(* Logix 5000 Program export KEP; software revision 30.00; part 10 of 15 *)

ADD_ON_INSTRUCTION L_CLR   (* revision 1.0 20170709, vendor Ken Fischer, NSWCPD, C516 *)
// CLR (64-bit)
// Revision note:
// Initial Release
// Help:
// Adds two LINT (signed 64-bit) values and returns a LINT (signed 64-bit) sum.
// Also provides math status bits for Carry, Negative, Overflow and Zero result
// (equivalent to built-in S:C, S:N, S:V, S:Z).
VAR_IN_OUT
   Out : LINT; {required}   // Sum, 64-bit Integer
END_VAR
VAR
   Wrk : DINT[2];   // Input A as two 32-bit DINTs
END_VAR

ROUTINE Logic   (* ladder *)
// Do 64-bit addition
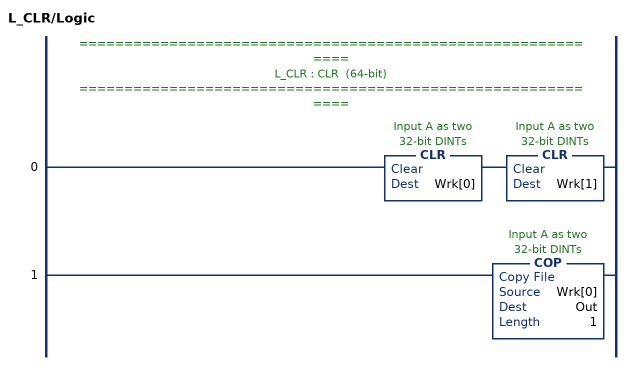
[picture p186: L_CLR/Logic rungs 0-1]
   // ============================================================
   // L_CLR : CLR  (64-bit)
   // ============================================================
   0: CLR(Wrk[0])CLR(Wrk[1]);
   1: COP(Wrk[0],Out,1);
END_ROUTINE
END_ADD_ON_INSTRUCTION

ADD_ON_INSTRUCTION L_EQU   (* revision 1.0 01 Release, vendor Rockwell Automation, ExecuteEnableInFalse *)
// Equal (64-bit)
// Revision note:
// Deleted unused Local Tag
// Help:
// This instruction compares two LINT (64-bit signed integer) variables.
// If Inp_A is equal to Inp_B, EnableOut and Out are set to true (1).
// Otherwise EnableOut and Out are cleared to false (0).
VAR_IN_OUT
   Inp_A : LINT; {required}   // Input A
   Inp_B : LINT; {required}   // Input B
END_VAR
VAR_OUTPUT
   Out : BOOL; {access Read Only, visible}   // TRUE if Inp_A is greater than or equal to Inp_B
END_VAR
VAR
   Wrk_Inp_B : DINT[2];   // 32-bit portions of Input B
   Wrk_Inp_A : DINT[2];   // 32-bit portions of Input A
END_VAR

ROUTINE EnableInFalse   (* ladder *)
// If rung is false, clear output "Out"
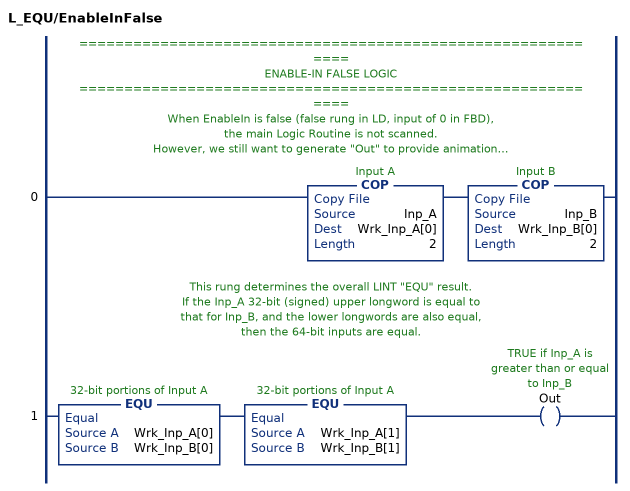
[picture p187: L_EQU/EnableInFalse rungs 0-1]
   // ============================================================
   // ENABLE-IN FALSE LOGIC
   // ============================================================
   // When EnableIn is false (false rung in LD, input of 0 in FBD),
   // the main Logic Routine is not scanned.
   // However, we still want to generate "Out" to provide animation!
   // ===================================================
   // CONVERT LINTs TO DINTs
   // ===================================================
   // These COPies take the input LINTs and break them into a
   // pair of DINTs each.  If the corresponding DINTs (high-order and high-order,
   // and low-order and low-order) are equal, then the input LINTs are equal.
   0: COP(Inp_A,Wrk_Inp_A[0],2)COP(Inp_B,Wrk_Inp_B[0],2);
   // This rung determines the overall LINT "EQU" result.
   // If the Inp_A 32-bit (signed) upper longword is equal to
   // that for Inp_B, and the lower longwords are also equal,
   // then the 64-bit inputs are equal.
   1: EQU(Wrk_Inp_A[0],Wrk_Inp_B[0])EQU(Wrk_Inp_A[1],Wrk_Inp_B[1])OTE(Out);
END_ROUTINE

ROUTINE Logic   (* ladder *)
// Compare inputs and output TRUE if they are equal
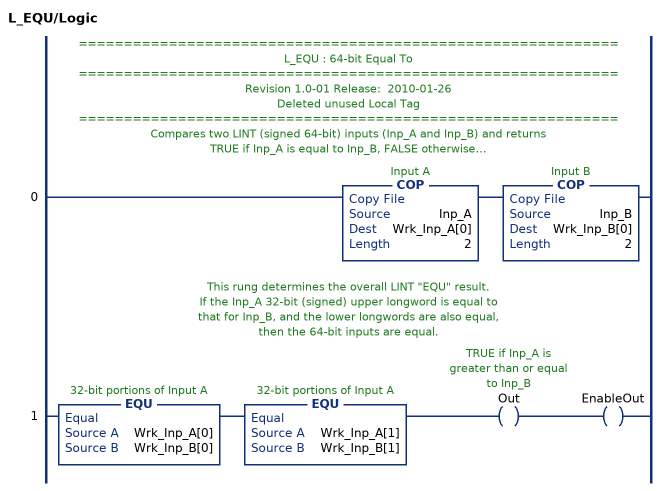
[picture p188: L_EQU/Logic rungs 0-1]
   // ============================================================
   // L_EQU : 64-bit Equal To
   // ============================================================
   // Revision 1.0-01 Release:  2010-01-26
   // Deleted unused Local Tag
   // ============================================================
   // Compares two LINT (signed 64-bit) inputs (Inp_A and Inp_B) and returns
   // TRUE if Inp_A is equal to Inp_B, FALSE otherwise.
   // This instruction breaks each LINT inputs into two DINTs
   // (32 bit signed each) to do the comparison.
   // ===================================================
   // CONVERT LINTs TO DINTs
   // ===================================================
   // These COPies take the input LINTs and break them into a
   // pair of DINTs each.  If the corresponding DINTs (high-order and high-order,
   // and low-order and low-order) are equal, then the input LINTs are equal.
   0: COP(Inp_A,Wrk_Inp_A[0],2)COP(Inp_B,Wrk_Inp_B[0],2);
   // This rung determines the overall LINT "EQU" result.
   // If the Inp_A 32-bit (signed) upper longword is equal to
   // that for Inp_B, and the lower longwords are also equal,
   // then the 64-bit inputs are equal.
   1: EQU(Wrk_Inp_A[0],Wrk_Inp_B[0])EQU(Wrk_Inp_A[1],Wrk_Inp_B[1])OTE(Out)OTE(EnableOut);
END_ROUTINE
END_ADD_ON_INSTRUCTION

ADD_ON_INSTRUCTION L_LES   (* revision 1.1 20170624, vendor Ken Fischer, NSWCPD, C516, ExecuteEnableInFalse *)
// Less Than (64-bit)
// Revision note:
// Rev1.1:  20170624 - Corrected comment on the Out bit
// Help:
// This instruction compares two LINT (64-bit signed integer) variables.
// If Inp_A is less than Inp_B, EnableOut and Out are set to true (1).
// Otherwise EnableOut and Out are cleared to false (0).
VAR_IN_OUT
   Inp_A : LINT; {required}   // Input A
   Inp_B : LINT; {required}   // Input B
END_VAR
VAR_OUTPUT
   Out : BOOL; {access Read Only, visible}   // TRUE if Inp_A is less than Inp_B
END_VAR
VAR
   Wrk_Inp_B : DINT[4];   // 32-bit portions of Input B
   Wrk_Inp_A : DINT[4];   // 32-bit portions of Input A
END_VAR

ROUTINE EnableInFalse   (* ladder *)
// If rung is false, clear output "Out"
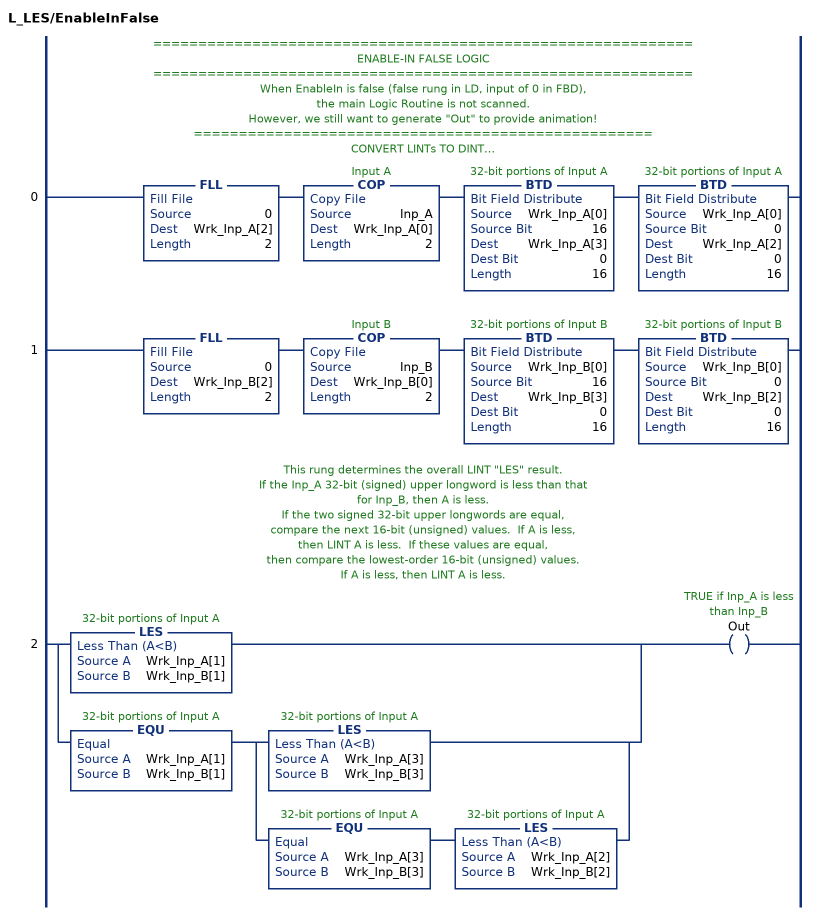
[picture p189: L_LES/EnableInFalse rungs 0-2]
   // ============================================================
   // ENABLE-IN FALSE LOGIC
   // ============================================================
   // When EnableIn is false (false rung in LD, input of 0 in FBD),
   // the main Logic Routine is not scanned.
   // However, we still want to generate "Out" to provide animation!
   // ===================================================
   // CONVERT LINTs TO DINTs
   // ===================================================
   // These COPies and BTDs take the input LINTs and break them into a
   // pair of DINTs each, then take the low-order signed DINT and breaks it
   // further into two 16-bit values so we can do unsigned compares on them.
   // Logix V17 has a LINT data type, but math instructions
   // (and AOI Input and Output Parameters) don't support LINT.
   0: FLL(0,Wrk_Inp_A[2],2)COP(Inp_A,Wrk_Inp_A[0],2)BTD(Wrk_Inp_A[0],16,Wrk_Inp_A[3],0,16)BTD(Wrk_Inp_A[0],0,Wrk_Inp_A[2],0,16);
   1: FLL(0,Wrk_Inp_B[2],2)COP(Inp_B,Wrk_Inp_B[0],2)BTD(Wrk_Inp_B[0],16,Wrk_Inp_B[3],0,16)BTD(Wrk_Inp_B[0],0,Wrk_Inp_B[2],0,16);
   // This rung determines the overall LINT "LES" result.
   // If the Inp_A 32-bit (signed) upper longword is less than that
   // for Inp_B, then A is less.
   // If the two signed 32-bit upper longwords are equal,
   // compare the next 16-bit (unsigned) values.  If A is less,
   // then LINT A is less.  If these values are equal,
   // then compare the lowest-order 16-bit (unsigned) values.
   // If A is less, then LINT A is less.
   2: [LES(Wrk_Inp_A[1],Wrk_Inp_B[1]) ,EQU(Wrk_Inp_A[1],Wrk_Inp_B[1]) [LES(Wrk_Inp_A[3],Wrk_Inp_B[3]) ,EQU(Wrk_Inp_A[3],Wrk_Inp_B[3]) LES(Wrk_Inp_A[2],Wrk_Inp_B[2]) ] ]OTE(Out);
END_ROUTINE

ROUTINE Logic   (* ladder *)
// Compare inputs and output TRUE if Inp_A < Inp_B
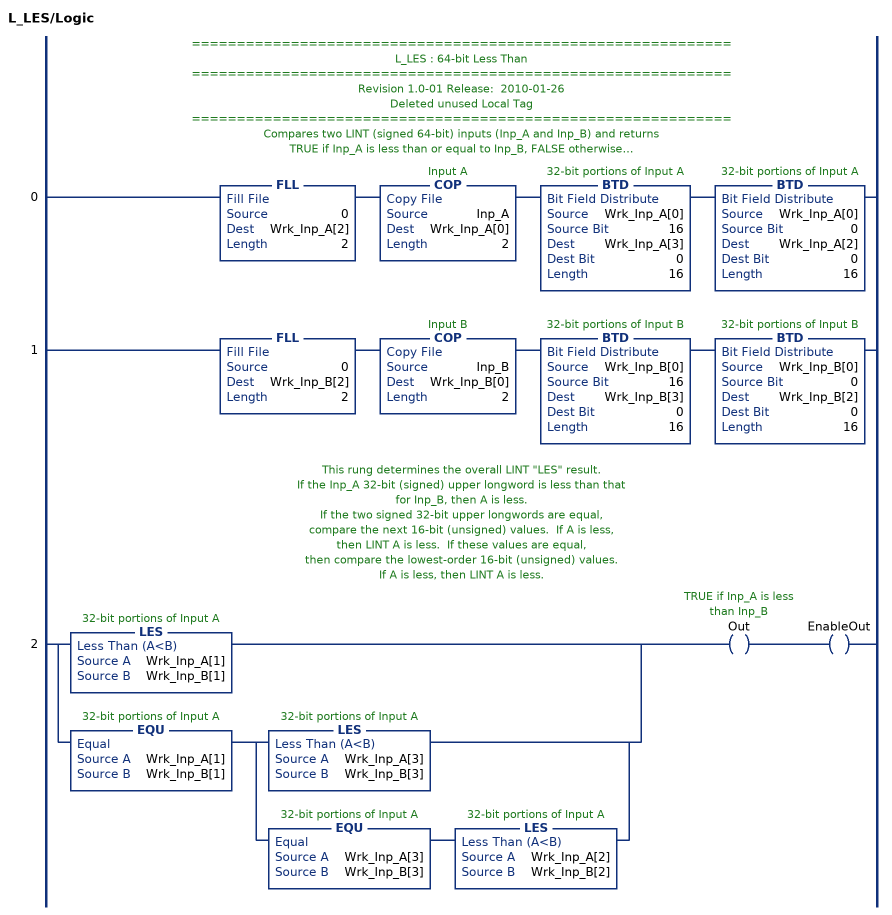
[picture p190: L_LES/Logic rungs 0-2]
   // ============================================================
   // L_LES : 64-bit Less Than
   // ============================================================
   // Revision 1.0-01 Release:  2010-01-26
   // Deleted unused Local Tag
   // ============================================================
   // Compares two LINT (signed 64-bit) inputs (Inp_A and Inp_B) and returns
   // TRUE if Inp_A is less than or equal to Inp_B, FALSE otherwise.
   // This instruction breaks the LINT inputs into three DINTs
   // (32 bit signed, 16 bit unsigned and 16 bit unsigned) to do the comparison.
   // ===================================================
   // CONVERT LINTs TO DINTs
   // ===================================================
   // These COPies and BTDs take the input LINTs and break them into a
   // pair of DINTs each, then take the low-order signed DINT and breaks it
   // further into two 16-bit values so we can do unsigned compares on them.
   // Logix V17 has a LINT data type, but math instructions
   // (and AOI Input and Output Parameters) don't support LINT.
   0: FLL(0,Wrk_Inp_A[2],2)COP(Inp_A,Wrk_Inp_A[0],2)BTD(Wrk_Inp_A[0],16,Wrk_Inp_A[3],0,16)BTD(Wrk_Inp_A[0],0,Wrk_Inp_A[2],0,16);
   1: FLL(0,Wrk_Inp_B[2],2)COP(Inp_B,Wrk_Inp_B[0],2)BTD(Wrk_Inp_B[0],16,Wrk_Inp_B[3],0,16)BTD(Wrk_Inp_B[0],0,Wrk_Inp_B[2],0,16);
   // This rung determines the overall LINT "LES" result.
   // If the Inp_A 32-bit (signed) upper longword is less than that
   // for Inp_B, then A is less.
   // If the two signed 32-bit upper longwords are equal,
   // compare the next 16-bit (unsigned) values.  If A is less,
   // then LINT A is less.  If these values are equal,
   // then compare the lowest-order 16-bit (unsigned) values.
   // If A is less, then LINT A is less.
   2: [LES(Wrk_Inp_A[1],Wrk_Inp_B[1]) ,EQU(Wrk_Inp_A[1],Wrk_Inp_B[1]) [LES(Wrk_Inp_A[3],Wrk_Inp_B[3]) ,EQU(Wrk_Inp_A[3],Wrk_Inp_B[3]) LES(Wrk_Inp_A[2],Wrk_Inp_B[2]) ] ]OTE(Out)OTE(EnableOut);
END_ROUTINE
END_ADD_ON_INSTRUCTION

ADD_ON_INSTRUCTION L_GRT   (* revision 1.0 01 Release, vendor Rockwell Automation, ExecuteEnableInFalse *)
// Greater Than (64-bit)
// Revision note:
// Deleted unused Local Tag
// Help:
// This instruction compares two LINT (64-bit signed integer) variables.
// If Inp_A is greater than Inp_B, EnableOut and Out are set to true (1).
// Otherwise EnableOut and Out are cleared to false (0).
VAR_IN_OUT
   Inp_A : LINT; {required}   // Input A
   Inp_B : LINT; {required}   // Input B
END_VAR
VAR_OUTPUT
   Out : BOOL; {access Read Only, visible}   // TRUE if Inp_A is greater than Inp_B
END_VAR
VAR
   Wrk_Inp_B : DINT[4];   // 32-bit portions of Input B
   Wrk_Inp_A : DINT[4];   // 32-bit portions of Input A
END_VAR

ROUTINE EnableInFalse   (* ladder *)
// If rung is false, clear output "Out"
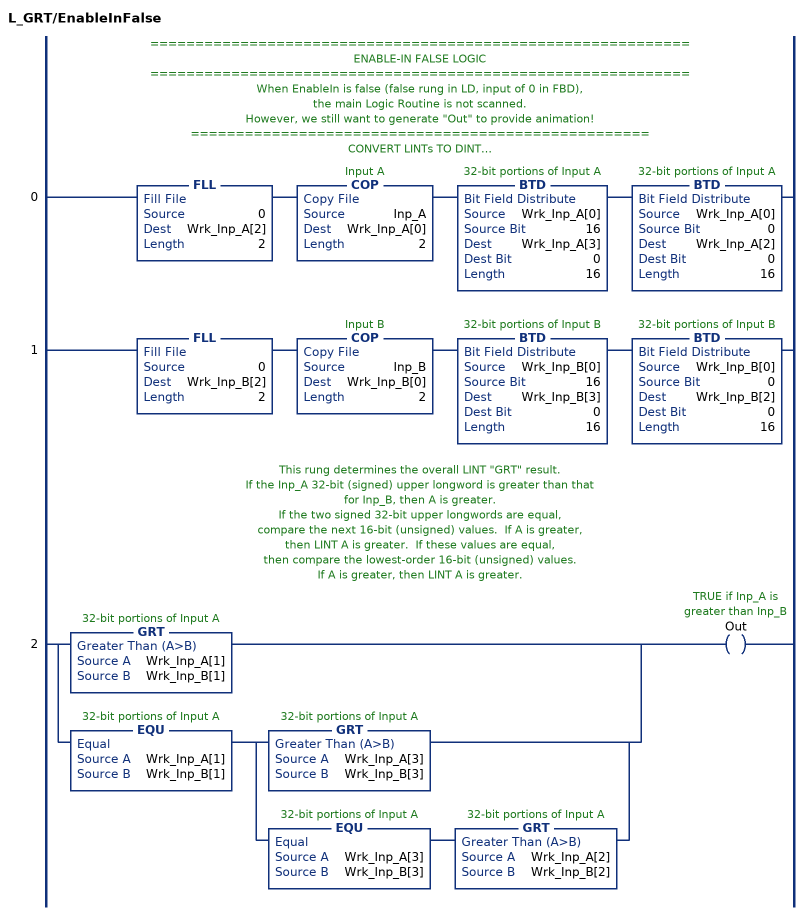
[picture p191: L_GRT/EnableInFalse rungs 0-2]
   // ============================================================
   // ENABLE-IN FALSE LOGIC
   // ============================================================
   // When EnableIn is false (false rung in LD, input of 0 in FBD),
   // the main Logic Routine is not scanned.
   // However, we still want to generate "Out" to provide animation!
   // ===================================================
   // CONVERT LINTs TO DINTs
   // ===================================================
   // These COPies and BTDs take the input LINTs and break them into a
   // pair of DINTs each, then take the low-order signed DINT and breaks it
   // further into two 16-bit values so we can do unsigned compares on them.
   // Logix V17 has a LINT data type, but math instructions
   // (and AOI Input and Output Parameters) don't support LINT.
   0: FLL(0,Wrk_Inp_A[2],2)COP(Inp_A,Wrk_Inp_A[0],2)BTD(Wrk_Inp_A[0],16,Wrk_Inp_A[3],0,16)BTD(Wrk_Inp_A[0],0,Wrk_Inp_A[2],0,16);
   1: FLL(0,Wrk_Inp_B[2],2)COP(Inp_B,Wrk_Inp_B[0],2)BTD(Wrk_Inp_B[0],16,Wrk_Inp_B[3],0,16)BTD(Wrk_Inp_B[0],0,Wrk_Inp_B[2],0,16);
   // This rung determines the overall LINT "GRT" result.
   // If the Inp_A 32-bit (signed) upper longword is greater than that
   // for Inp_B, then A is greater.
   // If the two signed 32-bit upper longwords are equal,
   // compare the next 16-bit (unsigned) values.  If A is greater,
   // then LINT A is greater.  If these values are equal,
   // then compare the lowest-order 16-bit (unsigned) values.
   // If A is greater, then LINT A is greater.
   2: [GRT(Wrk_Inp_A[1],Wrk_Inp_B[1]) ,EQU(Wrk_Inp_A[1],Wrk_Inp_B[1]) [GRT(Wrk_Inp_A[3],Wrk_Inp_B[3]) ,EQU(Wrk_Inp_A[3],Wrk_Inp_B[3]) GRT(Wrk_Inp_A[2],Wrk_Inp_B[2]) ] ]OTE(Out);
END_ROUTINE

ROUTINE Logic   (* ladder *)
// Compare inputs and output TRUE if Inp_A > Inp_B
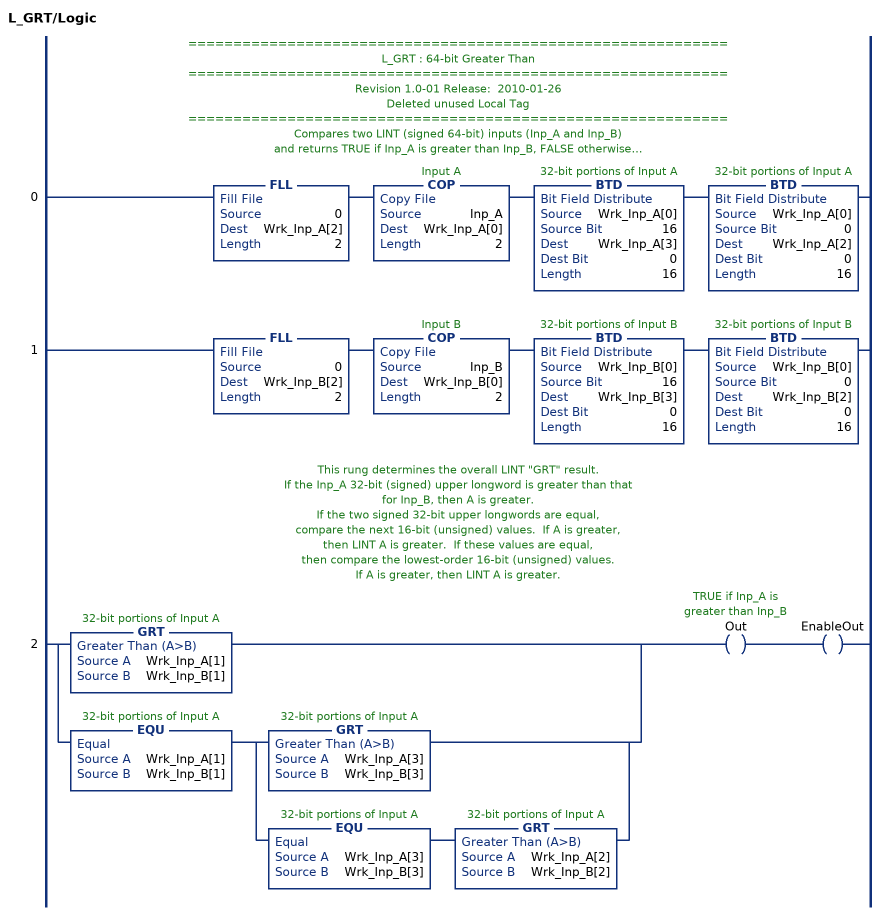
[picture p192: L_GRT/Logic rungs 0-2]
   // ============================================================
   // L_GRT : 64-bit Greater Than
   // ============================================================
   // Revision 1.0-01 Release:  2010-01-26
   // Deleted unused Local Tag
   // ============================================================
   // Compares two LINT (signed 64-bit) inputs (Inp_A and Inp_B)
   // and returns TRUE if Inp_A is greater than Inp_B, FALSE otherwise.
   // This instruction breaks the LINT inputs into three DINTs
   // (32 bit signed, 16 bit unsigned and 16 bit unsigned) to do the comparison.
   // ===================================================
   // CONVERT LINTs TO DINTs
   // ===================================================
   // These COPies and BTDs take the input LINTs and break them into a
   // pair of DINTs each, then take the low-order signed DINT and breaks it
   // further into two 16-bit values so we can do unsigned compares on them.
   // Logix V17 has a LINT data type, but math instructions
   // (and AOI Input and Output Parameters) don't support LINT.
   0: FLL(0,Wrk_Inp_A[2],2)COP(Inp_A,Wrk_Inp_A[0],2)BTD(Wrk_Inp_A[0],16,Wrk_Inp_A[3],0,16)BTD(Wrk_Inp_A[0],0,Wrk_Inp_A[2],0,16);
   1: FLL(0,Wrk_Inp_B[2],2)COP(Inp_B,Wrk_Inp_B[0],2)BTD(Wrk_Inp_B[0],16,Wrk_Inp_B[3],0,16)BTD(Wrk_Inp_B[0],0,Wrk_Inp_B[2],0,16);
   // This rung determines the overall LINT "GRT" result.
   // If the Inp_A 32-bit (signed) upper longword is greater than that
   // for Inp_B, then A is greater.
   // If the two signed 32-bit upper longwords are equal,
   // compare the next 16-bit (unsigned) values.  If A is greater,
   // then LINT A is greater.  If these values are equal,
   // then compare the lowest-order 16-bit (unsigned) values.
   // If A is greater, then LINT A is greater.
   2: [GRT(Wrk_Inp_A[1],Wrk_Inp_B[1]) ,EQU(Wrk_Inp_A[1],Wrk_Inp_B[1]) [GRT(Wrk_Inp_A[3],Wrk_Inp_B[3]) ,EQU(Wrk_Inp_A[3],Wrk_Inp_B[3]) GRT(Wrk_Inp_A[2],Wrk_Inp_B[2]) ] ]OTE(Out)OTE(EnableOut);
END_ROUTINE
END_ADD_ON_INSTRUCTION

ADD_ON_INSTRUCTION L_MOV   (* revision 1.0 20170709, vendor Ken Fischer, NSWCPD, C516 *)
// MOV (64-bit)
// Revision note:
// Initial Release
// Help:
// Adds two LINT (signed 64-bit) values and returns a LINT (signed 64-bit) sum.
// Also provides math status bits for Carry, Negative, Overflow and Zero result
// (equivalent to built-in S:C, S:N, S:V, S:Z).
VAR_IN_OUT
   Inp : LINT; {required}   // First Addend, 64-bit Integer
   Out : LINT; {required}   // Sum, 64-bit Integer
END_VAR
VAR
   Wrk : DINT[2];   // Input A as two 32-bit DINTs
END_VAR

ROUTINE Logic   (* ladder *)
// Do 64-bit addition
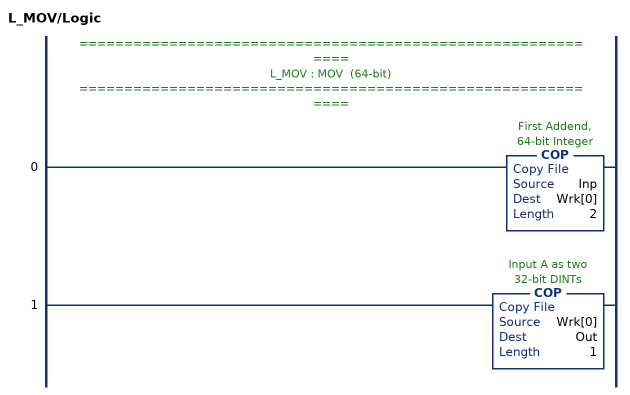
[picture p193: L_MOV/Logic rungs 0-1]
   // ============================================================
   // L_MOV : MOV  (64-bit)
   // ============================================================
   0: COP(Inp,Wrk[0],2);
   1: COP(Wrk[0],Out,1);
END_ROUTINE
END_ADD_ON_INSTRUCTION

VAR_GLOBAL   (* controller tags *)
   EdDSA_KS : DINT[8];
   EdDSA_KS_Prime : DINT[8];
   EdDSA_MSG_FROM_NODE1 : EdDSA_MSG;
   EdDSA_MSG_FROM_NODE2 : EdDSA_MSG := (Status.RunMode := 1); {consumed}
        ConsumeInfo(Producer := NODE2, RemoteTag := EdDSA_MSG_TO_NODE1, RemoteInstance := 0, RPI := 20)
   EdDSA_MSG_FROM_NODE3 : EdDSA_MSG := (Status.RunMode := 1); {consumed}
        ConsumeInfo(Producer := NODE3, RemoteTag := EdDSA_MSG_TO_NODE1, RemoteInstance := 0, RPI := 20)
   EdDSA_MSG_FROM_NODE4 : EdDSA_MSG := (Status.RunMode := 1); {consumed}
        ConsumeInfo(Producer := NODE4, RemoteTag := EdDSA_MSG_TO_NODE1, RemoteInstance := 0, RPI := 20)
   EdDSA_MSG_NODE_BLANK : EdDSA_MSG;
   EdDSA_MSG_TO_NODE1 : EdDSA_MSG := (Status.RunMode := 1); {produced}
        ProduceInfo(ProduceCount := 1)
   EdDSA_MSG_TO_NODE2 : EdDSA_MSG := (Status.RunMode := 1, Flags := 807424, KsID := 884046357013193, KsPrimeID := 884046357013193, Counter := 2, Sig_R := 'd364eff9ccfcc97018fd0ba62d4a326842ebc7d4f48434492f5901a5f45a3cdc', Sig_S := 'd25f2cd9950480b758ba73154021eaf02fe75d547178015ecae934d14dc91302'); {produced}
        ProduceInfo(ProduceCount := 1)
   EdDSA_MSG_TO_NODE3 : EdDSA_MSG := (Status.RunMode := 1, Flags := 807424, KsID := 884046357013193, KsPrimeID := 884046357013193, Counter := 2, Sig_R := 'd364eff9ccfcc97018fd0ba62d4a326842ebc7d4f48434492f5901a5f45a3cdc', Sig_S := 'd25f2cd9950480b758ba73154021eaf02fe75d547178015ecae934d14dc91302'); {produced}
        ProduceInfo(ProduceCount := 1)
   EdDSA_MSG_TO_NODE4 : EdDSA_MSG := (Status.RunMode := 1, Flags := 807424, KsID := 884040507585218, KsPrimeID := 884040507585218, Counter := 1, Sig_R := '324bd46bf27b6cb22cee8aa952b18efd33700e928981e6a429b187bfc86ab21b', Sig_S := '65b33a1798ff6af8ec3cf5e2754cfa862b3e0157dbcf5aaa4cf57b46265abe04'); {produced}
        ProduceInfo(ProduceCount := 1)
   FirstScan_EdDSA : BOOL;
   InternalFlag_AllNodesHaveMyKs : BOOL;
   InternalFlag_AllNodesHaveMyKsPrime : BOOL;
   InternalFlag_KsID : LINT;
   InternalFlag_KsPrimeID : LINT;
   NODE : VMAC_DATA_INTERNAL[5];
   Wrk_InpA : DINT[2];
   Wrk_InpB : DINT[2];
END_VAR

PROGRAM KEP   (* main routine MainRoutine *)
VAR
   B256_COMPARE : B256_COMPARE;
   B256_CtoE : B256_CtoE;
   B256_CtoS : B256_CtoS;
   B256_DINTtoE : B256_DINTtoE;
   B256_EtoC : B256_EtoC;
   B256_EtoDINT : B256_EtoDINT;
   B256_EtoL : B256_EtoL;
   B256_StoC : B256_StoC;
   B256_StoC_LE : B256_StoC_LE;
   B256_StoSLE : B256_StoSLE;
   Ed25519_SIGN1 : Ed25519_SIGN := (SEQCTRL_DN := 1);
   Ed25519_SIGN2 : Ed25519_SIGN := (SEQCTRL_DN := 1);
   Ed25519_SIGN3 : Ed25519_SIGN := (SEQCTRL_DN := 1);
   Ed25519_SIGN4 : Ed25519_SIGN := (SEQCTRL_DN := 1);
   Ed25519_VERIFY : Ed25519_VERIFY := (Out_Status := 666, SEQCTRL_DN := 1);
   EdDSA_INTERNAL : EdDSA_INTERNAL[5] := ([2].MsgCopy.Status.RunMode := 1, [2].MsgToBeVerified.Status.RunMode := 1, [2].VerificationStatus := 666, [3].MsgCopy.Status.RunMode := 1, [3].VerificationStatus := 666, [4].MsgCopy.Status.RunMode := 1, [4].VerificationStatus := 666);
        [1].MSGLASTVERIFIED.FLAGS.9   // Ks' Available
        [1].MSGLASTVERIFIED.FLAGS.12   // Ks = Ks' Status
        [2].MSGTOBEVERIFIED.FLAGS.3   // EdDH Key Pair Available
        [2].MSGTOBEVERIFIED.FLAGS.7   // Ks' Request
        [2].MSGTOBEVERIFIED.FLAGS.14   // Key Server Yes
        [2].MSGTOBEVERIFIED.FLAGS.15   // Key Server No
        [2].MSGLASTVERIFIED.FLAGS.3   // EdDH Public Value Available
        [2].MSGLASTVERIFIED.FLAGS.7   // Ks' Request
        [2].MSGLASTVERIFIED.FLAGS.9   // Ks' Available
        [2].MSGLASTVERIFIED.FLAGS.12   // Ks = Ks' Status
        [2].MSGLASTVERIFIED.FLAGS.14   // Key Server Yes
        [2].MSGLASTVERIFIED.FLAGS.15   // Key Server No
        [3].MSGLASTVERIFIED.FLAGS.9   // Ks' Available
        [3].MSGLASTVERIFIED.FLAGS.12   // Ks = Ks' Status
        [4].MSGLASTVERIFIED.FLAGS.9   // Ks' Available
        [4].MSGLASTVERIFIED.FLAGS.12   // Ks = Ks' Status
   EdDSA_INTERNAL_PublicKeys : STRING[5] := ([1] := '0c9a8de38256c73f37c6b288fdbb2056f321e1265e57f29f23378dd0b1e66638', [2] := 'e1ac8af046694475b0f6e4e8c6fc5f48f66bcfdda71f7fe253a0c9939196a19b', [3] := 'd654f92efff5cea22a438e8516cc8a0cb3ece216582c390773c420b5fcba85a4', [4] := '3f54436d46973deca0dd68b3ff830c052ec91fcb1ea3b590f74077c541452ba4');
   EdDSA_STATES : EdDSA_STATECTRL[15] := ([0].TIMER[1].PRE := 1200000, [1].TIMER[1].PRE := 600000, ...);
   InternalFlags : InternalFlags[5];
        [0]   // BLANK
   InternalFlag_AllNodesUsingKsPrime : BOOL;
   InternalFlag_ALLOK : BOOL;
   InternalFlag_CreateNewKsPrime : BOOL;
   InternalFlag_KeyServerIdentityNo : BOOL;
   InternalFlag_KeyServerIdentityYes : BOOL;
   InternalFlag_KsEqualKsPrimeStatus : BOOL;
   InternalFlag_KsExists : BOOL;
   InternalFlag_KsIDMatchesServer : BOOL;
   InternalFlag_KsPrimeAvail : BOOL;
   InternalFlag_KsPrimeExists : BOOL;
   InternalFlag_KsPrimeIDMatchesServer : BOOL;
   InternalFlag_PowerOnCycle : BOOL;
   Internal_EdDSA_Msg : EdDSA_MSG := (Flags := 807424, KsID := 884046357013193, KsPrimeID := 884046357013193, Counter := 2, Sig_R := 'd364eff9ccfcc97018fd0ba62d4a326842ebc7d4f48434492f5901a5f45a3cdc', Sig_S := 'd25f2cd9950480b758ba73154021eaf02fe75d547178015ecae934d14dc91302');
   Internal_PriKeyPrefix : STRING := '24841cb5d01820bfedf3dbc329d8566e72647164af40cf7093d786602b8f7350';
   Internal_PriKeyScalar : STRING := '693652680d76c4f31c5ba156e5091eb5b49492b8a2414c632f8d0bfbfdbfeab0';
   Internal_PubKey : STRING := '0c9a8de38256c73f37c6b288fdbb2056f321e1265e57f29f23378dd0b1e66638';
   KAF_REMOVEME : BOOL;
   KsPrimeExchangeErrorTimer : TIMER := (PRE := 3000);
   ListenerDelayTimer : TIMER := (PRE := 60000);
   L_CLR : L_CLR;
   L_GRT : L_GRT;
   L_MOV : L_MOV;
   MainVerifyQue : DINT;
   MSG_ADDR : STRING;
   MyNodeNumber : DINT := 1;
   POINT_DEC : POINT_DEC;
   POINT_ENC : POINT_ENC;
   POINT_MUL : POINT_MUL;
   PRN : STRING := 'e2550481408387bd8839935086ca31d50421d03a173d9e68d88aee87dbdec183';
   PRNG : PRNG := (SEQCTRL_DN := 1);
   PRNG_Constant : STRING := 'ade0423dfbca187338137abcdef0123456789abcdef0123456789abc0deaabdc';
   PRNG_Counter : LINT := 7;
   PRNG_Seed : LINT[13] := ([0] := 4901681123204320363, [1] := -632144198763559951, [2] := 2976335046112202042, [3] := 8288841210875444234, [4] := 9167634160563233835, [5] := 37532181834330076, [6] := -2856874913592792556, [7] := -6349952886226467258, [8] := 6332976598348069210, [9] := -5196275024322241072, [10] := -6128352333910660567, [11] := 6023154382974024002, [12] := 2114970212779298212);
   ProcessorState : DINT;
   ServerNode : INT := 1;
   ServerPriority : DINT[5] := ([1] := 1, [2] := 2, [3] := 3, [4] := 4);
   SHA512_SEQ : SHA512_SEQ := (Inp_LEN := 4);
   SignedMsgDest : INT;   // 0=None 1=Server 2=Client 3=All
   Temp_Listener_C1 : DINT[22];
   Temp_Listener_C10 : DINT[22];
   Temp_Listener_C11 : DINT[22];
   Temp_Listener_C12 : DINT[22] := ([0] := 1);
   Temp_Listener_C2 : DINT[22];
   Temp_Listener_C3 : DINT[22];
   Temp_Listener_C4 : DINT[22];
   Temp_Listener_C5 : DINT[22];
   Temp_Listener_C6 : DINT[22];
   Temp_Listener_C7 : DINT[22];
   Temp_Listener_C8 : DINT[22];
   Temp_Listener_C9 : DINT[22];
   Temp_Listener_D1 : DINT[43];
   Temp_Listener_D2 : DINT[43];
   Temp_Listener_E1 : DINT[32];
   Temp_Listener_E2 : DINT[32];
   Temp_Listener_E3 : DINT[32];
   Temp_Listener_HASH : LINT[8] := ([0] := 4806167800202152510, [1] := 3888285838775000601, [2] := -140984029611778028, [3] := 1946554300050844520, [4] := 5363287658015379789, [5] := 3226180144845580150, [6] := -3663149285472923576, [7] := 7971327916595242900);
   Temp_Listener_L : LINT[4] := ([0] := 3096980842655755, [1] := 49551693482492080, [2] := 792827095719873280, [3] := -5761510542191579125);
   Temp_Listener_MSG : LINT[1600];
   Temp_Listener_P1 : POINT := (X[0] := 1306, X[1] := 605, X[2] := 143, X[3] := 726, X[4] := 2390, X[5] := 2860, X[6] := 1447, X[7] := 2386, X[8] := 1888, X[9] := 716, X[10] := 3177, X[11] := 3525, X[12] := 3542, X[13] := 799, X[14] := 1250, X[15] := 3082, X[16] := 1022, X[17] := 1765, X[18] := 973, X[19] := 877, X[20] := 361, X[21] := 2, Y[0] := 1624, Y[1] := 1638, Y[2] := 1638, Y[3] := 1638, Y[4] := 1638, Y[5] := 1638, Y[6] := 1638, Y[7] := 1638, Y[8] := 1638, Y[9] := 1638, Y[10] := 1638, Y[11] := 1638, Y[12] := 1638, Y[13] := 1638, Y[14] := 1638, Y[15] := 1638, Y[16] := 1638, Y[17] := 1638, Y[18] := 1638, Y[19] := 1638, Y[20] := 1638, Y[21] := 6, Z[0] := 1);
   Temp_Listener_P2 : POINT;
   Temp_Listener_P3 : POINT;
   Temp_Listener_P4 : POINT;
   Temp_Processor_C1 : DINT[22];
   Temp_Processor_C10 : DINT[22];
   Temp_Processor_C11 : DINT[22];
   Temp_Processor_C12 : DINT[22];
   Temp_Processor_C2 : DINT[22];
   Temp_Processor_C3 : DINT[22];
   Temp_Processor_C4 : DINT[22];
   Temp_Processor_C5 : DINT[22];
   Temp_Processor_C6 : DINT[22];
   Temp_Processor_C7 : DINT[22];
   Temp_Processor_C8 : DINT[22];
   Temp_Processor_C9 : DINT[22];
   Temp_Processor_D1 : DINT[43];
   Temp_Processor_D2 : DINT[43];
   Temp_Processor_DINT1 : DINT[8];
   Temp_Processor_DINT2 : DINT[8];
   Temp_Processor_E1 : DINT[32];
   Temp_Processor_E2 : DINT[32];
   Temp_Processor_E3 : DINT[32];
   Temp_Processor_HASH : LINT[8] := ([0] := 1656079617683781305, [1] := -585368191651055373, [2] := -8735768536564435700, [3] := -7848544442316980786, [4] := 64937589855949566, [5] := -6375838580187852433, [6] := -6442917330651579307, [7] := -335753469374272444);
   Temp_Processor_L : LINT[4] := ([0] := 2252349703749640, [1] := 36037595259994240, [2] := 576601524159907840, [3] := -9221119687151026168);
   Temp_Processor_MSG : LINT[1600];
   Temp_Processor_P1 : POINT := (X[0] := 1306, X[1] := 605, X[2] := 143, X[3] := 726, X[4] := 2390, X[5] := 2860, X[6] := 1447, X[7] := 2386, X[8] := 1888, X[9] := 716, X[10] := 3177, X[11] := 3525, X[12] := 3542, X[13] := 799, X[14] := 1250, X[15] := 3082, X[16] := 1022, X[17] := 1765, X[18] := 973, X[19] := 877, X[20] := 361, X[21] := 2, Y[0] := 1624, Y[1] := 1638, Y[2] := 1638, Y[3] := 1638, Y[4] := 1638, Y[5] := 1638, Y[6] := 1638, Y[7] := 1638, Y[8] := 1638, Y[9] := 1638, Y[10] := 1638, Y[11] := 1638, Y[12] := 1638, Y[13] := 1638, Y[14] := 1638, Y[15] := 1638, Y[16] := 1638, Y[17] := 1638, Y[18] := 1638, Y[19] := 1638, Y[20] := 1638, Y[21] := 6, Z[0] := 1);
   Temp_Processor_P2 : POINT;
   Temp_Processor_P3 : POINT;
   Temp_Processor_P4 : POINT;
   Temp_Processor_S : STRING := '0213c94dd134e9ca5e017871545de72ff0ea21401573ba58b7800495d92c5fd2';
   T_DINT1 : DINT;
   T_DINT2 : DINT;
   T_INT1 : INT := 64;
   VerificationInProgress : BOOL;
   VerifyNextServing : DINT;
   VerifyNode : DINT := 4;
   VerifyOneshot : BOOL := 1;
   VerifyQueTemp : DINT := 666;
   WorkingNode : DINT;
END_VAR

ROUTINE LISTENER   (* ladder *)
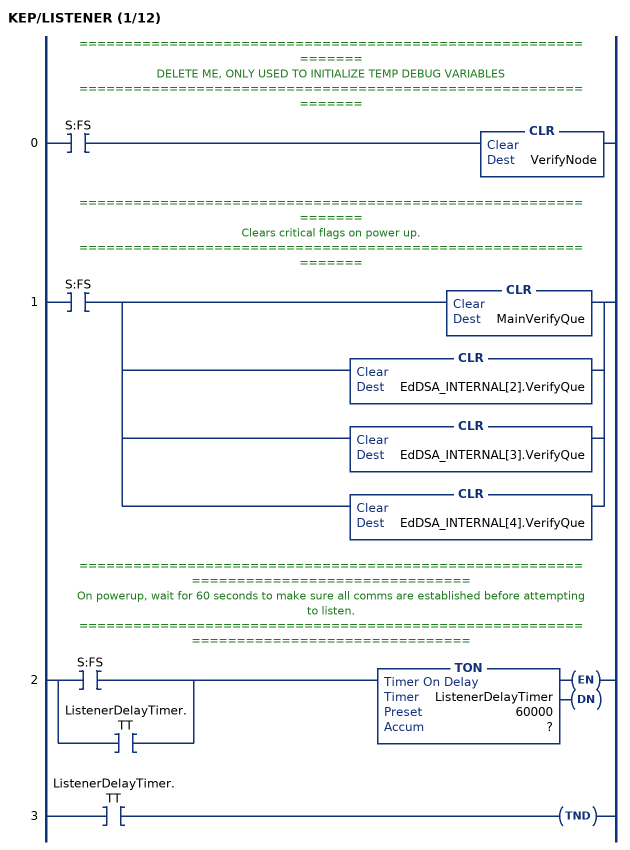
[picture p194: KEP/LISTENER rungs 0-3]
   // ===============================================================
   // DELETE ME, ONLY USED TO INITIALIZE TEMP DEBUG VARIABLES
   // ===============================================================
   0: XIC(S:FS)CLR(VerifyNode);
   // ===============================================================
   // Clears critical flags on power up.
   // ===============================================================
   1: XIC(S:FS)[CLR(MainVerifyQue) ,CLR(EdDSA_INTERNAL[2].VerifyQue) ,CLR(EdDSA_INTERNAL[3].VerifyQue) ,CLR(EdDSA_INTERNAL[4].VerifyQue) ];
   // =======================================================================================
   // On powerup, wait for 60 seconds to make sure all comms are established before attempting to listen.
   // =======================================================================================
   2: [XIC(S:FS) ,XIC(ListenerDelayTimer.TT) ]TON(ListenerDelayTimer,?,?);
   3: XIC(ListenerDelayTimer.TT)TND();
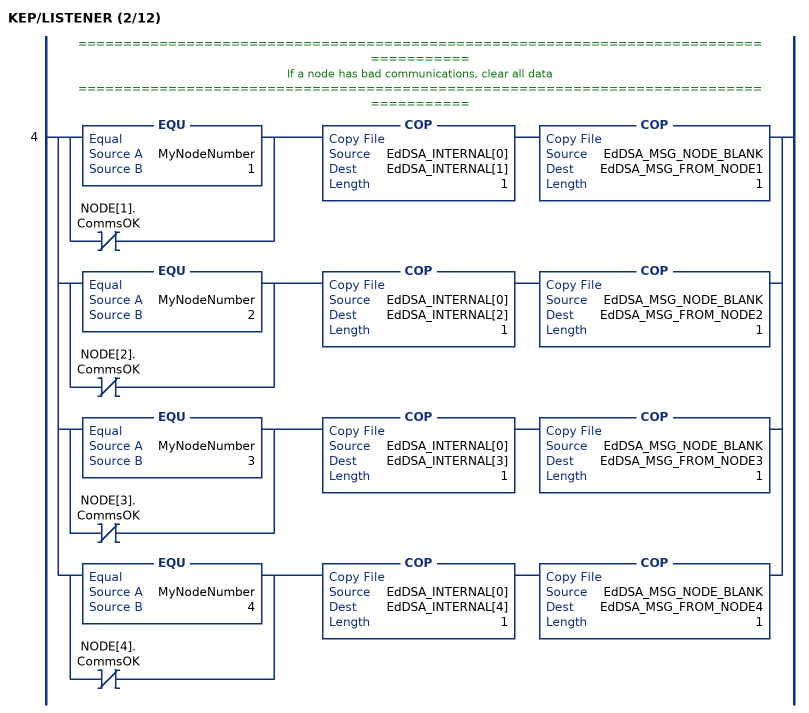
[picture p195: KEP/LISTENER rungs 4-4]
   // =======================================================================================
   // If a node has bad communications, clear all data
   // =======================================================================================
   4: [[EQU(MyNodeNumber,1) ,XIO(NODE[1].CommsOK) ] COP(EdDSA_INTERNAL[0],EdDSA_INTERNAL[1],1) COP(EdDSA_MSG_NODE_BLANK,EdDSA_MSG_FROM_NODE1,1) ,[EQU(MyNodeNumber,2) ,XIO(NODE[2].CommsOK) ] COP(EdDSA_INTERNAL[0],EdDSA_INTERNAL[2],1) COP(EdDSA_MSG_NODE_BLANK,EdDSA_MSG_FROM_NODE2,1) ,[EQU(MyNodeNumber,3) ,XIO(NODE[3].CommsOK) ] COP(EdDSA_INTERNAL[0],EdDSA_INTERNAL[3],1) COP(EdDSA_MSG_NODE_BLANK,EdDSA_MSG_FROM_NODE3,1) ,[EQU(MyNodeNumber,4) ,XIO(NODE[4].CommsOK) ] COP(EdDSA_INTERNAL[0],EdDSA_INTERNAL[4],1) COP(EdDSA_MSG_NODE_BLANK,EdDSA_MSG_FROM_NODE4,1) ];
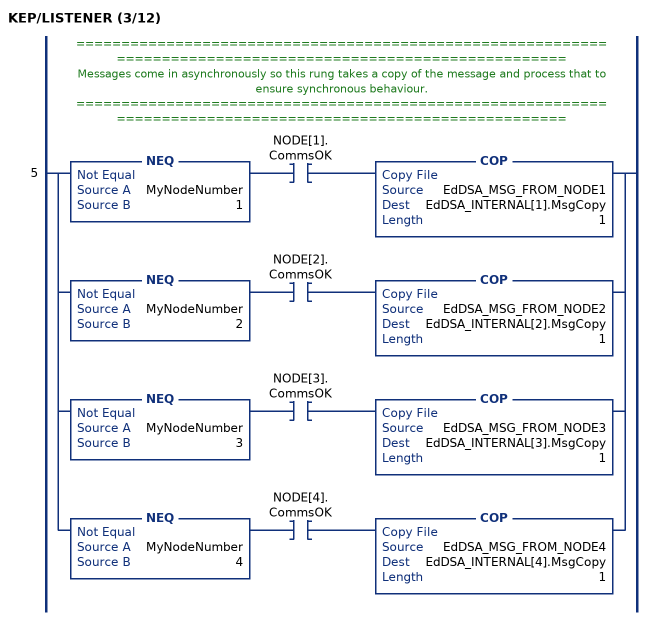
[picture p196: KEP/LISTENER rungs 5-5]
   // =============================================================================================================
   // Messages come in asynchronously so this rung takes a copy of the message and process that to ensure synchronous behaviour.
   // =============================================================================================================
   5: [NEQ(MyNodeNumber,1) XIC(NODE[1].CommsOK) COP(EdDSA_MSG_FROM_NODE1,EdDSA_INTERNAL[1].MsgCopy,1) ,NEQ(MyNodeNumber,2) XIC(NODE[2].CommsOK) COP(EdDSA_MSG_FROM_NODE2,EdDSA_INTERNAL[2].MsgCopy,1) ,NEQ(MyNodeNumber,3) XIC(NODE[3].CommsOK) COP(EdDSA_MSG_FROM_NODE3,EdDSA_INTERNAL[3].MsgCopy,1) ,NEQ(MyNodeNumber,4) XIC(NODE[4].CommsOK) COP(EdDSA_MSG_FROM_NODE4,EdDSA_INTERNAL[4].MsgCopy,1) ];
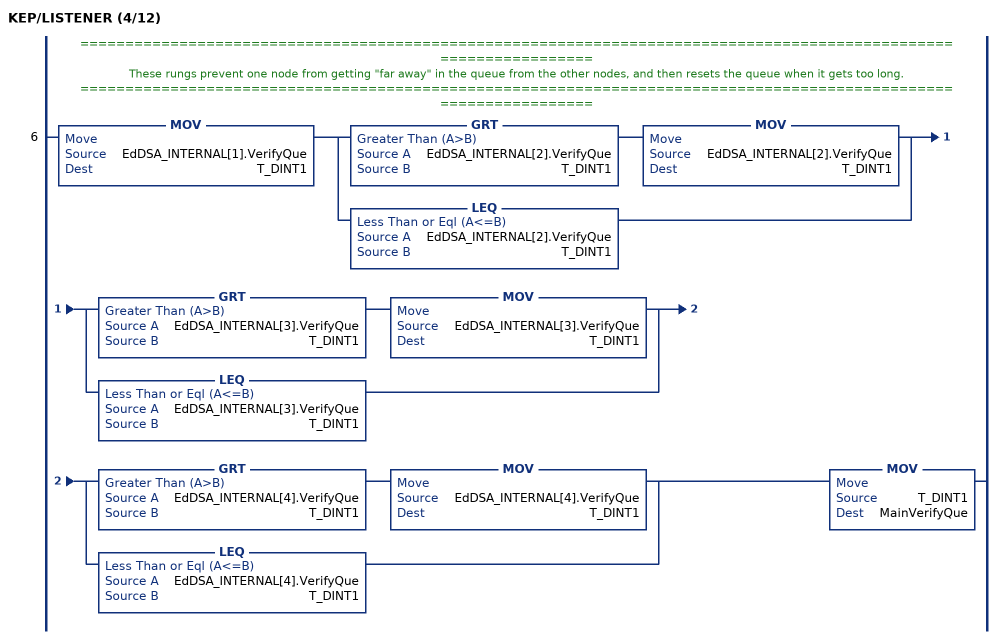
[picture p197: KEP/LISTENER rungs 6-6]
   // ==================================================================================================================
   // These rungs prevent one node from getting "far away" in the queue from the other nodes, and then resets the queue when it gets too long.
   // ==================================================================================================================
   6: MOV(EdDSA_INTERNAL[1].VerifyQue,T_DINT1)[GRT(EdDSA_INTERNAL[2].VerifyQue,T_DINT1) MOV(EdDSA_INTERNAL[2].VerifyQue,T_DINT1) ,LEQ(EdDSA_INTERNAL[2].VerifyQue,T_DINT1) ][GRT(EdDSA_INTERNAL[3].VerifyQue,T_DINT1) MOV(EdDSA_INTERNAL[3].VerifyQue,T_DINT1) ,LEQ(EdDSA_INTERNAL[3].VerifyQue,T_DINT1) ][GRT(EdDSA_INTERNAL[4].VerifyQue,T_DINT1) MOV(EdDSA_INTERNAL[4].VerifyQue,T_DINT1) ,LEQ(EdDSA_INTERNAL[4].VerifyQue,T_DINT1) ]MOV(T_DINT1,MainVerifyQue);
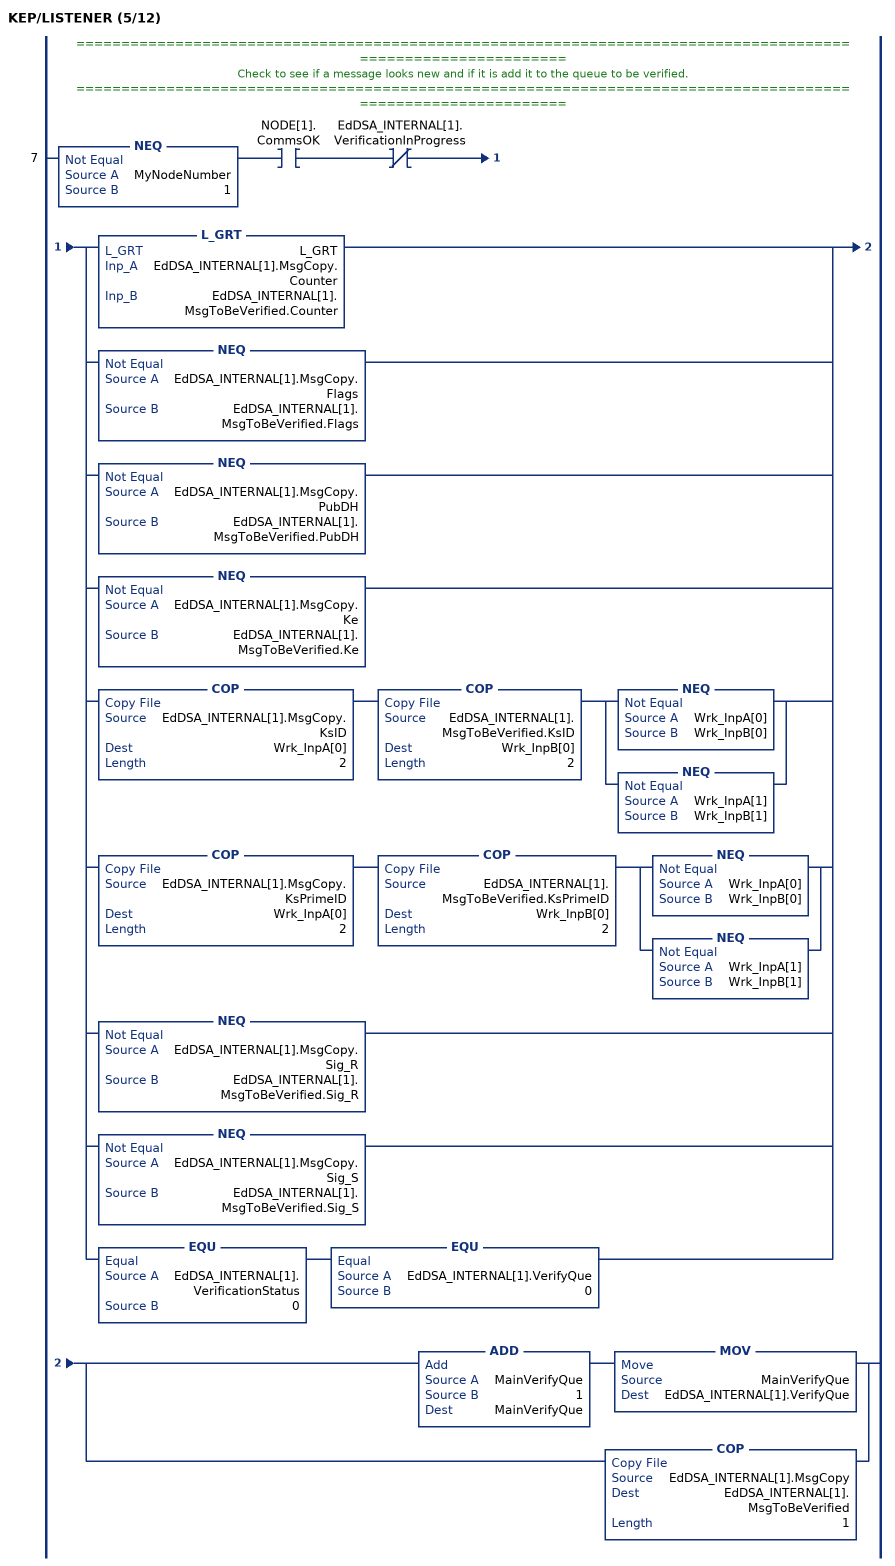
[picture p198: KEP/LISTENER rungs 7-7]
   // =============================================================================================================
   // Check to see if a message looks new and if it is add it to the queue to be verified.
   // =============================================================================================================
   7: NEQ(MyNodeNumber,1)XIC(NODE[1].CommsOK)XIO(EdDSA_INTERNAL[1].VerificationInProgress)[L_GRT(L_GRT,EdDSA_INTERNAL[1].MsgCopy.Counter,EdDSA_INTERNAL[1].MsgToBeVerified.Counter) ,NEQ(EdDSA_INTERNAL[1].MsgCopy.Flags,EdDSA_INTERNAL[1].MsgToBeVerified.Flags) ,NEQ(EdDSA_INTERNAL[1].MsgCopy.PubDH,EdDSA_INTERNAL[1].MsgToBeVerified.PubDH) ,NEQ(EdDSA_INTERNAL[1].MsgCopy.Ke,EdDSA_INTERNAL[1].MsgToBeVerified.Ke) ,COP(EdDSA_INTERNAL[1].MsgCopy.KsID,Wrk_InpA[0],2) COP(EdDSA_INTERNAL[1].MsgToBeVerified.KsID,Wrk_InpB[0],2) [NEQ(Wrk_InpA[0],Wrk_InpB[0]) ,NEQ(Wrk_InpA[1],Wrk_InpB[1]) ] ,COP(EdDSA_INTERNAL[1].MsgCopy.KsPrimeID,Wrk_InpA[0],2) COP(EdDSA_INTERNAL[1].MsgToBeVerified.KsPrimeID,Wrk_InpB[0],2) [NEQ(Wrk_InpA[0],Wrk_InpB[0]) ,NEQ(Wrk_InpA[1],Wrk_InpB[1]) ] ,NEQ(EdDSA_INTERNAL[1].MsgCopy.Sig_R,EdDSA_INTERNAL[1].MsgToBeVerified.Sig_R) ,NEQ(EdDSA_INTERNAL[1].MsgCopy.Sig_S,EdDSA_INTERNAL[1].MsgToBeVerified.Sig_S) ,EQU(EdDSA_INTERNAL[1].VerificationStatus,0) EQU(EdDSA_INTERNAL[1].VerifyQue,0) ][ADD(MainVerifyQue,1,MainVerifyQue) MOV(MainVerifyQue,EdDSA_INTERNAL[1].VerifyQue) ,COP(EdDSA_INTERNAL[1].MsgCopy,EdDSA_INTERNAL[1].MsgToBeVerified,1) ];
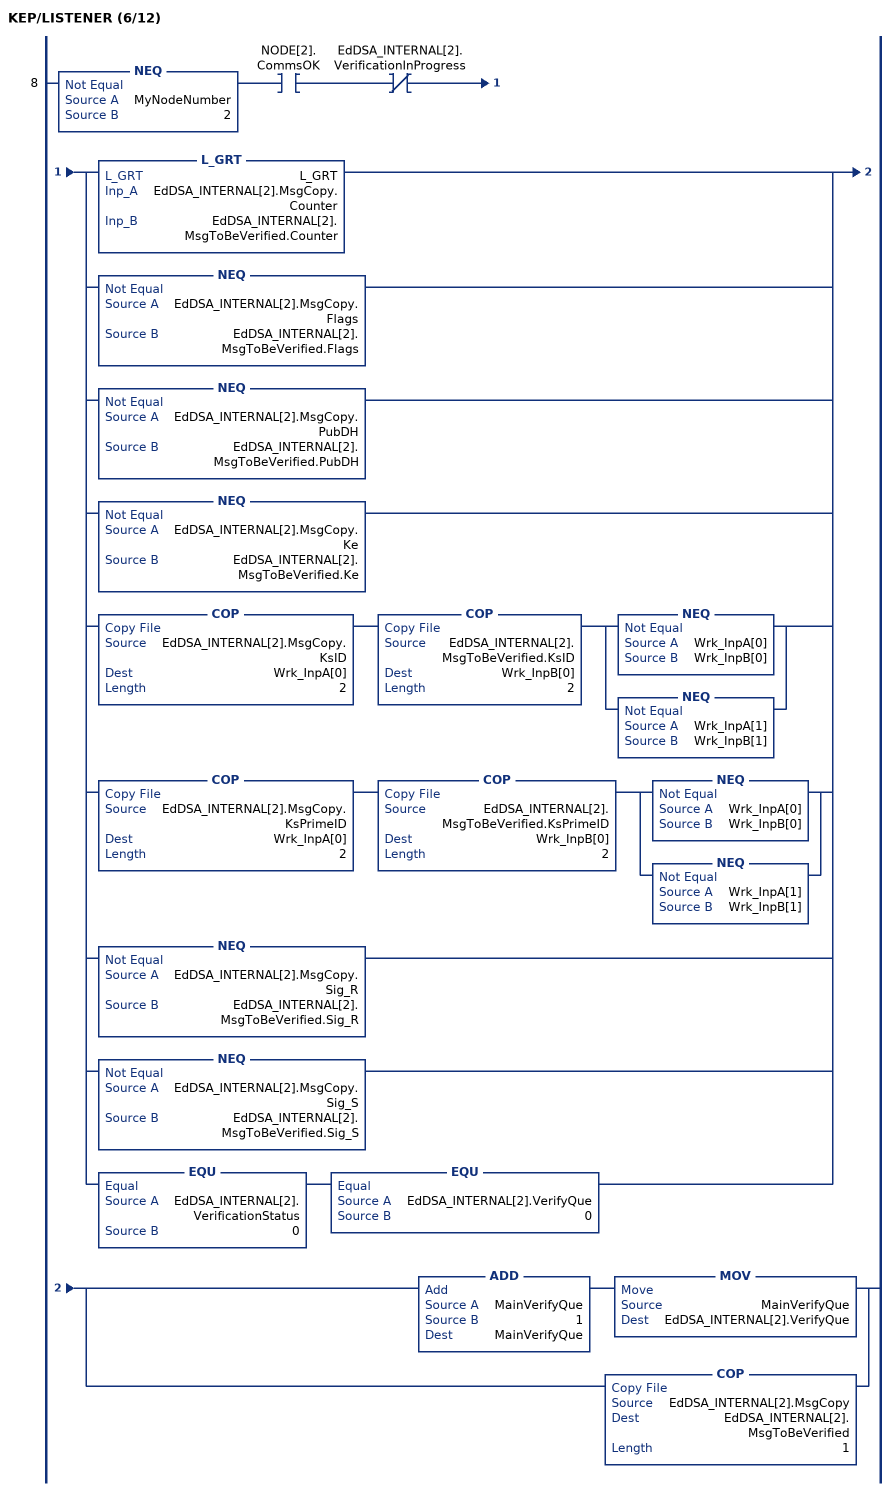
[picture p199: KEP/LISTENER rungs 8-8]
   8: NEQ(MyNodeNumber,2)XIC(NODE[2].CommsOK)XIO(EdDSA_INTERNAL[2].VerificationInProgress)[L_GRT(L_GRT,EdDSA_INTERNAL[2].MsgCopy.Counter,EdDSA_INTERNAL[2].MsgToBeVerified.Counter) ,NEQ(EdDSA_INTERNAL[2].MsgCopy.Flags,EdDSA_INTERNAL[2].MsgToBeVerified.Flags) ,NEQ(EdDSA_INTERNAL[2].MsgCopy.PubDH,EdDSA_INTERNAL[2].MsgToBeVerified.PubDH) ,NEQ(EdDSA_INTERNAL[2].MsgCopy.Ke,EdDSA_INTERNAL[2].MsgToBeVerified.Ke) ,COP(EdDSA_INTERNAL[2].MsgCopy.KsID,Wrk_InpA[0],2) COP(EdDSA_INTERNAL[2].MsgToBeVerified.KsID,Wrk_InpB[0],2) [NEQ(Wrk_InpA[0],Wrk_InpB[0]) ,NEQ(Wrk_InpA[1],Wrk_InpB[1]) ] ,COP(EdDSA_INTERNAL[2].MsgCopy.KsPrimeID,Wrk_InpA[0],2) COP(EdDSA_INTERNAL[2].MsgToBeVerified.KsPrimeID,Wrk_InpB[0],2) [NEQ(Wrk_InpA[0],Wrk_InpB[0]) ,NEQ(Wrk_InpA[1],Wrk_InpB[1]) ] ,NEQ(EdDSA_INTERNAL[2].MsgCopy.Sig_R,EdDSA_INTERNAL[2].MsgToBeVerified.Sig_R) ,NEQ(EdDSA_INTERNAL[2].MsgCopy.Sig_S,EdDSA_INTERNAL[2].MsgToBeVerified.Sig_S) ,EQU(EdDSA_INTERNAL[2].VerificationStatus,0) EQU(EdDSA_INTERNAL[2].VerifyQue,0) ][ADD(MainVerifyQue,1,MainVerifyQue) MOV(MainVerifyQue,EdDSA_INTERNAL[2].VerifyQue) ,COP(EdDSA_INTERNAL[2].MsgCopy,EdDSA_INTERNAL[2].MsgToBeVerified,1) ];
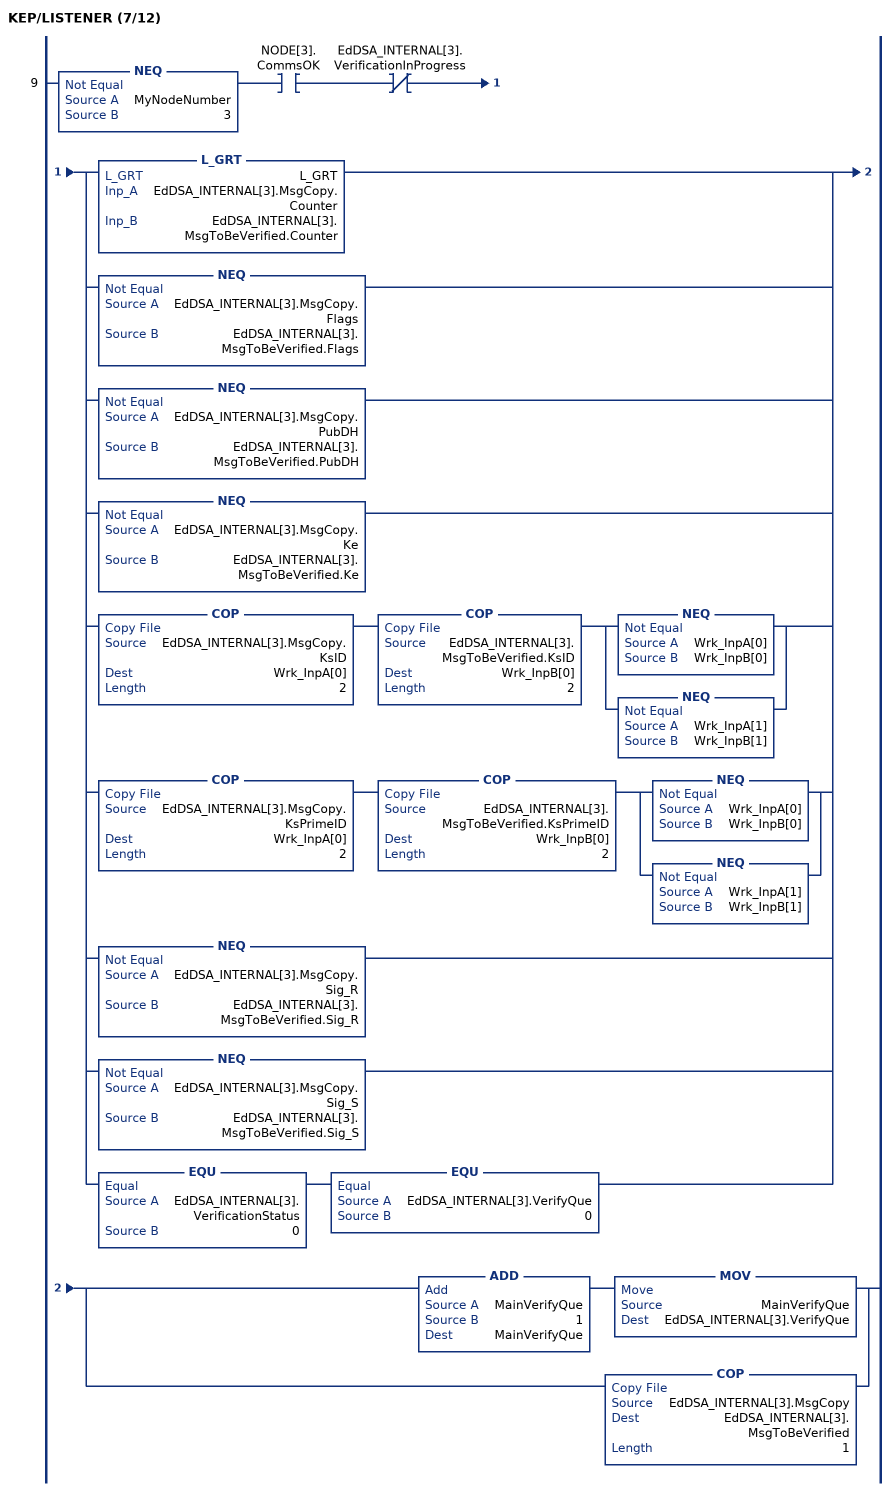
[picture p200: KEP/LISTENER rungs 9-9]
   9: NEQ(MyNodeNumber,3)XIC(NODE[3].CommsOK)XIO(EdDSA_INTERNAL[3].VerificationInProgress)[L_GRT(L_GRT,EdDSA_INTERNAL[3].MsgCopy.Counter,EdDSA_INTERNAL[3].MsgToBeVerified.Counter) ,NEQ(EdDSA_INTERNAL[3].MsgCopy.Flags,EdDSA_INTERNAL[3].MsgToBeVerified.Flags) ,NEQ(EdDSA_INTERNAL[3].MsgCopy.PubDH,EdDSA_INTERNAL[3].MsgToBeVerified.PubDH) ,NEQ(EdDSA_INTERNAL[3].MsgCopy.Ke,EdDSA_INTERNAL[3].MsgToBeVerified.Ke) ,COP(EdDSA_INTERNAL[3].MsgCopy.KsID,Wrk_InpA[0],2) COP(EdDSA_INTERNAL[3].MsgToBeVerified.KsID,Wrk_InpB[0],2) [NEQ(Wrk_InpA[0],Wrk_InpB[0]) ,NEQ(Wrk_InpA[1],Wrk_InpB[1]) ] ,COP(EdDSA_INTERNAL[3].MsgCopy.KsPrimeID,Wrk_InpA[0],2) COP(EdDSA_INTERNAL[3].MsgToBeVerified.KsPrimeID,Wrk_InpB[0],2) [NEQ(Wrk_InpA[0],Wrk_InpB[0]) ,NEQ(Wrk_InpA[1],Wrk_InpB[1]) ] ,NEQ(EdDSA_INTERNAL[3].MsgCopy.Sig_R,EdDSA_INTERNAL[3].MsgToBeVerified.Sig_R) ,NEQ(EdDSA_INTERNAL[3].MsgCopy.Sig_S,EdDSA_INTERNAL[3].MsgToBeVerified.Sig_S) ,EQU(EdDSA_INTERNAL[3].VerificationStatus,0) EQU(EdDSA_INTERNAL[3].VerifyQue,0) ][ADD(MainVerifyQue,1,MainVerifyQue) MOV(MainVerifyQue,EdDSA_INTERNAL[3].VerifyQue) ,COP(EdDSA_INTERNAL[3].MsgCopy,EdDSA_INTERNAL[3].MsgToBeVerified,1) ];
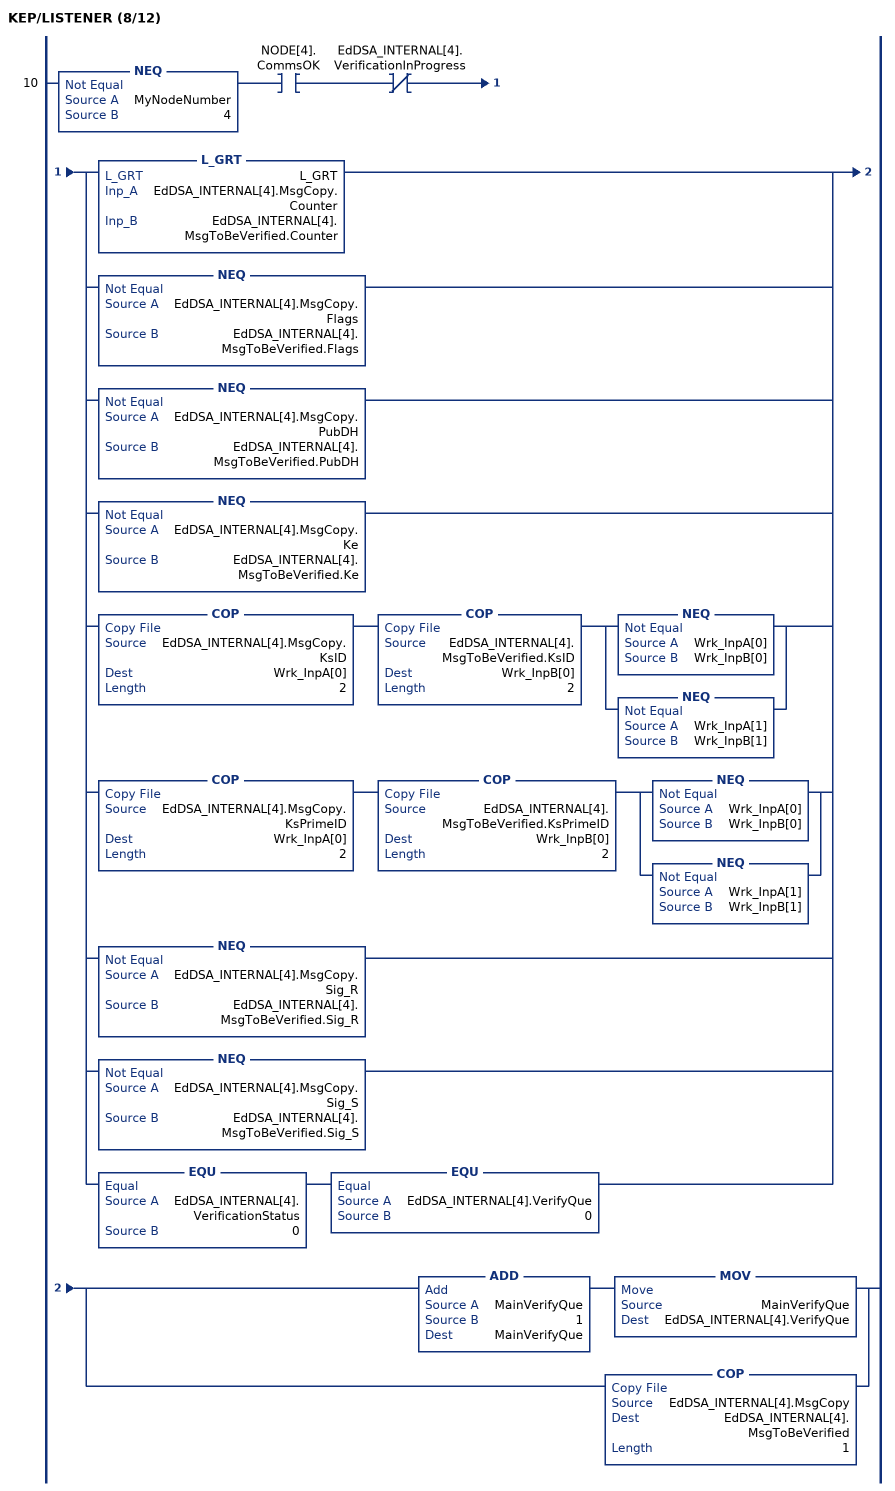
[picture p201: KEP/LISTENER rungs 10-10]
   10: NEQ(MyNodeNumber,4)XIC(NODE[4].CommsOK)XIO(EdDSA_INTERNAL[4].VerificationInProgress)[L_GRT(L_GRT,EdDSA_INTERNAL[4].MsgCopy.Counter,EdDSA_INTERNAL[4].MsgToBeVerified.Counter) ,NEQ(EdDSA_INTERNAL[4].MsgCopy.Flags,EdDSA_INTERNAL[4].MsgToBeVerified.Flags) ,NEQ(EdDSA_INTERNAL[4].MsgCopy.PubDH,EdDSA_INTERNAL[4].MsgToBeVerified.PubDH) ,NEQ(EdDSA_INTERNAL[4].MsgCopy.Ke,EdDSA_INTERNAL[4].MsgToBeVerified.Ke) ,COP(EdDSA_INTERNAL[4].MsgCopy.KsID,Wrk_InpA[0],2) COP(EdDSA_INTERNAL[4].MsgToBeVerified.KsID,Wrk_InpB[0],2) [NEQ(Wrk_InpA[0],Wrk_InpB[0]) ,NEQ(Wrk_InpA[1],Wrk_InpB[1]) ] ,COP(EdDSA_INTERNAL[4].MsgCopy.KsPrimeID,Wrk_InpA[0],2) COP(EdDSA_INTERNAL[4].MsgToBeVerified.KsPrimeID,Wrk_InpB[0],2) [NEQ(Wrk_InpA[0],Wrk_InpB[0]) ,NEQ(Wrk_InpA[1],Wrk_InpB[1]) ] ,NEQ(EdDSA_INTERNAL[4].MsgCopy.Sig_R,EdDSA_INTERNAL[4].MsgToBeVerified.Sig_R) ,NEQ(EdDSA_INTERNAL[4].MsgCopy.Sig_S,EdDSA_INTERNAL[4].MsgToBeVerified.Sig_S) ,EQU(EdDSA_INTERNAL[4].VerificationStatus,0) EQU(EdDSA_INTERNAL[4].VerifyQue,0) ][ADD(MainVerifyQue,1,MainVerifyQue) MOV(MainVerifyQue,EdDSA_INTERNAL[4].VerifyQue) ,COP(EdDSA_INTERNAL[4].MsgCopy,EdDSA_INTERNAL[4].MsgToBeVerified,1) ];
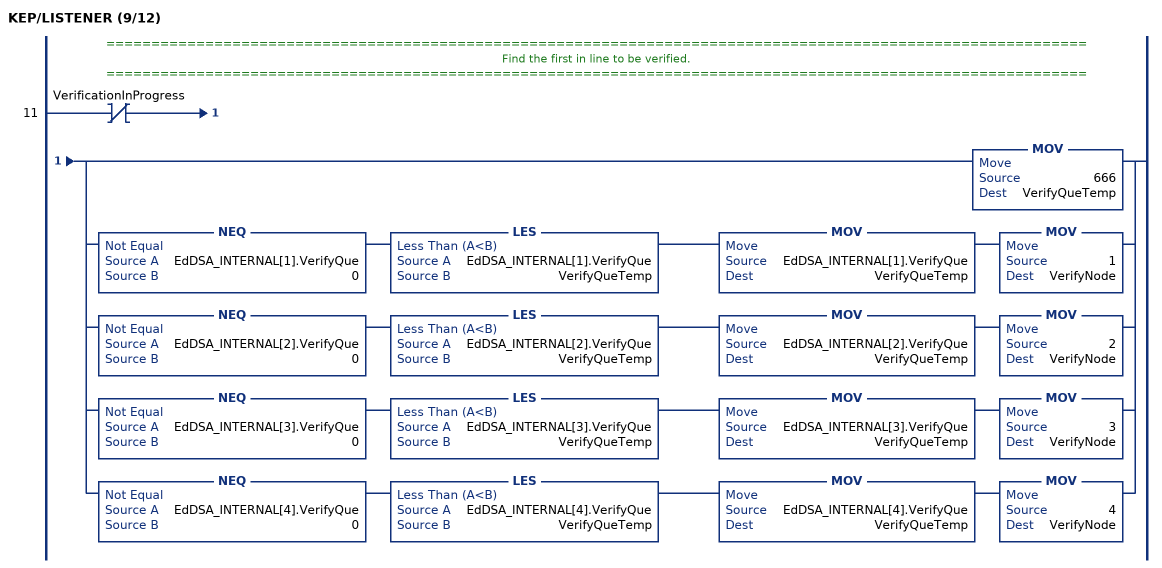
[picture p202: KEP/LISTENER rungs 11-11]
   // =============================================================================================================
   // Find the first in line to be verified.
   // =============================================================================================================
   11: XIO(VerificationInProgress)[MOV(666,VerifyQueTemp) ,NEQ(EdDSA_INTERNAL[1].VerifyQue,0) LES(EdDSA_INTERNAL[1].VerifyQue,VerifyQueTemp) MOV(EdDSA_INTERNAL[1].VerifyQue,VerifyQueTemp) MOV(1,VerifyNode) ,NEQ(EdDSA_INTERNAL[2].VerifyQue,0) LES(EdDSA_INTERNAL[2].VerifyQue,VerifyQueTemp) MOV(EdDSA_INTERNAL[2].VerifyQue,VerifyQueTemp) MOV(2,VerifyNode) ,NEQ(EdDSA_INTERNAL[3].VerifyQue,0) LES(EdDSA_INTERNAL[3].VerifyQue,VerifyQueTemp) MOV(EdDSA_INTERNAL[3].VerifyQue,VerifyQueTemp) MOV(3,VerifyNode) ,NEQ(EdDSA_INTERNAL[4].VerifyQue,0) LES(EdDSA_INTERNAL[4].VerifyQue,VerifyQueTemp) MOV(EdDSA_INTERNAL[4].VerifyQue,VerifyQueTemp) MOV(4,VerifyNode) ];
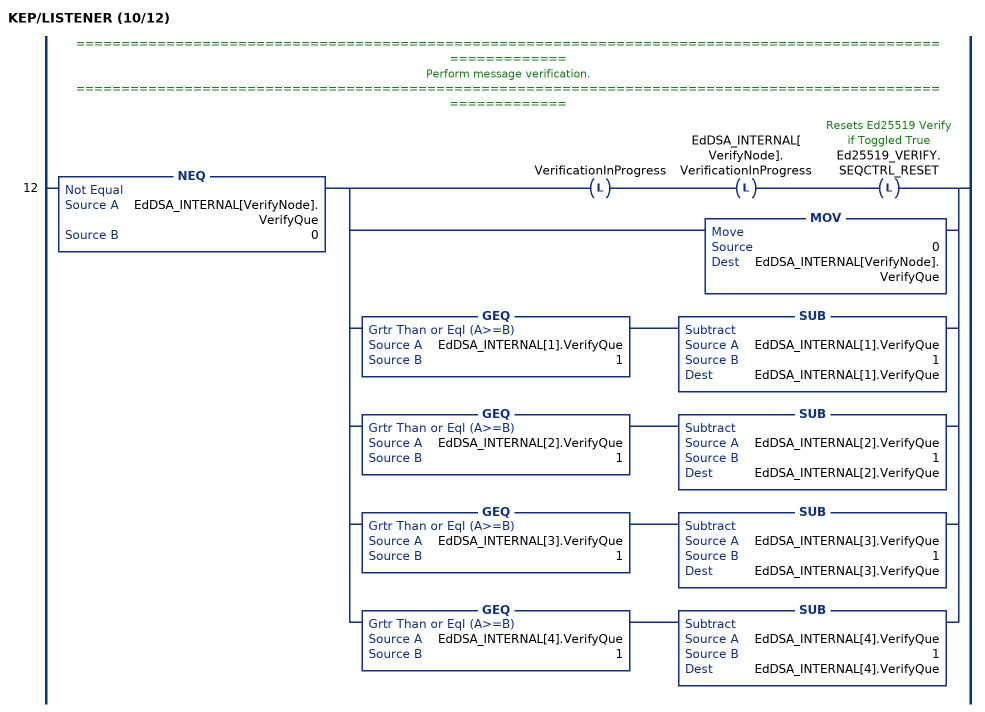
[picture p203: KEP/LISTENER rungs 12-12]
   // =============================================================================================================
   // Perform message verification.
   // =============================================================================================================
   12: NEQ(EdDSA_INTERNAL[VerifyNode].VerifyQue,0)[OTL(VerificationInProgress) OTL(EdDSA_INTERNAL[VerifyNode].VerificationInProgress) OTL(Ed25519_VERIFY.SEQCTRL_RESET) ,MOV(0,EdDSA_INTERNAL[VerifyNode].VerifyQue) ,GEQ(EdDSA_INTERNAL[1].VerifyQue,1) SUB(EdDSA_INTERNAL[1].VerifyQue,1,EdDSA_INTERNAL[1].VerifyQue) ,GEQ(EdDSA_INTERNAL[2].VerifyQue,1) SUB(EdDSA_INTERNAL[2].VerifyQue,1,EdDSA_INTERNAL[2].VerifyQue) ,GEQ(EdDSA_INTERNAL[3].VerifyQue,1) SUB(EdDSA_INTERNAL[3].VerifyQue,1,EdDSA_INTERNAL[3].VerifyQue) ,GEQ(EdDSA_INTERNAL[4].VerifyQue,1) SUB(EdDSA_INTERNAL[4].VerifyQue,1,EdDSA_INTERNAL[4].VerifyQue) ];
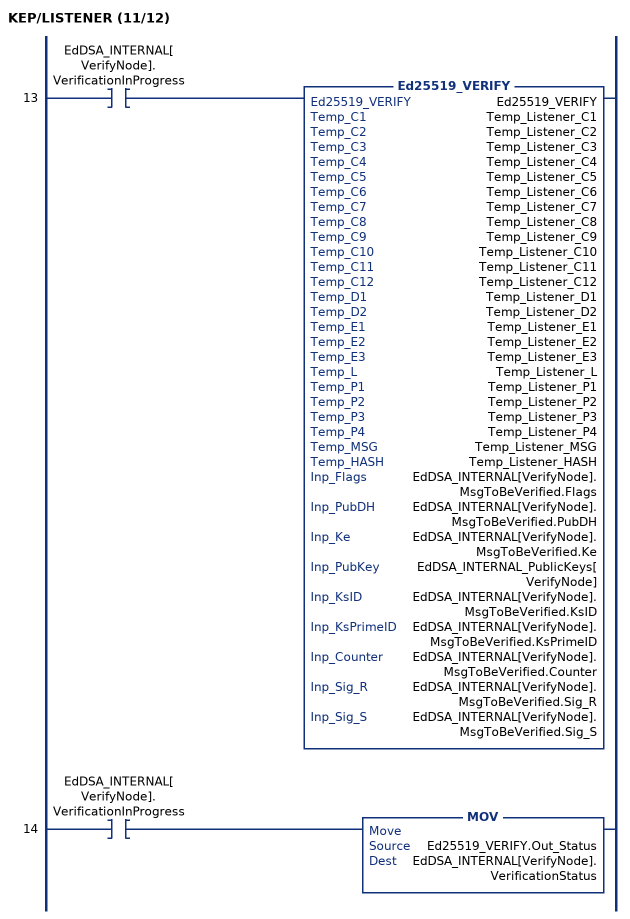
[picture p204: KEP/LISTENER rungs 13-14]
   13: XIC(EdDSA_INTERNAL[VerifyNode].VerificationInProgress)Ed25519_VERIFY(Ed25519_VERIFY,Temp_Listener_C1,Temp_Listener_C2,Temp_Listener_C3,Temp_Listener_C4,Temp_Listener_C5,Temp_Listener_C6,Temp_Listener_C7,Temp_Listener_C8,Temp_Listener_C9,Temp_Listener_C10,Temp_Listener_C11,Temp_Listener_C12,Temp_Listener_D1,Temp_Listener_D2,Temp_Listener_E1,Temp_Listener_E2,Temp_Listener_E3,Temp_Listener_L,Temp_Listener_P1,Temp_Listener_P2,Temp_Listener_P3,Temp_Listener_P4,Temp_Listener_MSG,Temp_Listener_HASH,EdDSA_INTERNAL[VerifyNode].MsgToBeVerified.Flags,EdDSA_INTERNAL[VerifyNode].MsgToBeVerified.PubDH,EdDSA_INTERNAL[VerifyNode].MsgToBeVerified.Ke,EdDSA_INTERNAL_PublicKeys[VerifyNode],EdDSA_INTERNAL[VerifyNode].MsgToBeVerified.KsID,EdDSA_INTERNAL[VerifyNode].MsgToBeVerified.KsPrimeID,EdDSA_INTERNAL[VerifyNode].MsgToBeVerified.Counter,EdDSA_INTERNAL[VerifyNode].MsgToBeVerified.Sig_R,EdDSA_INTERNAL[VerifyNode].MsgToBeVerified.Sig_S);
   14: XIC(EdDSA_INTERNAL[VerifyNode].VerificationInProgress)MOV(Ed25519_VERIFY.Out_Status,EdDSA_INTERNAL[VerifyNode].VerificationStatus);
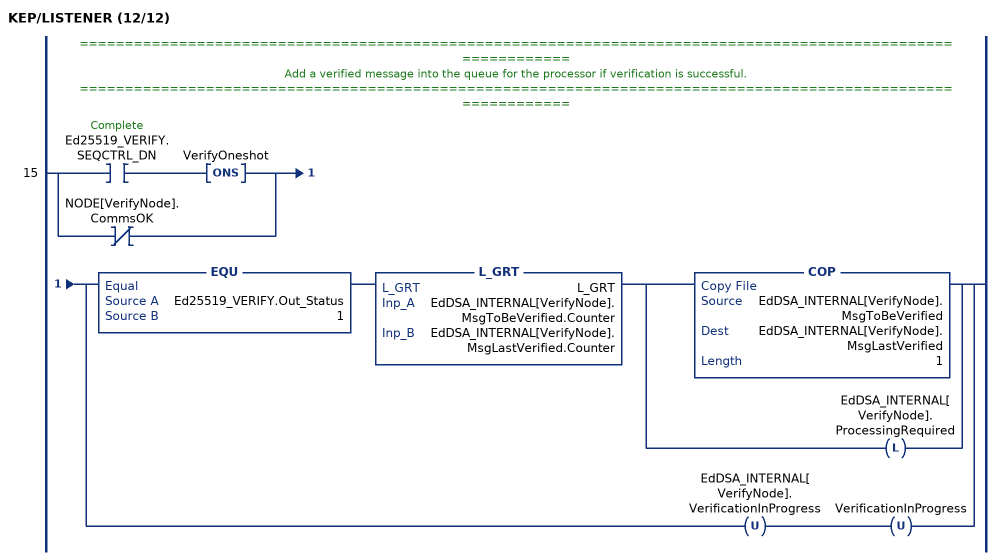
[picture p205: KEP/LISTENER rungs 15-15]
   // =============================================================================================================
   // Add a verified message into the queue for the processor if verification is successful.
   // =============================================================================================================
   15: [XIC(Ed25519_VERIFY.SEQCTRL_DN) ONS(VerifyOneshot) ,XIO(NODE[VerifyNode].CommsOK) ][EQU(Ed25519_VERIFY.Out_Status,1) L_GRT(L_GRT,EdDSA_INTERNAL[VerifyNode].MsgToBeVerified.Counter,EdDSA_INTERNAL[VerifyNode].MsgLastVerified.Counter) [COP(EdDSA_INTERNAL[VerifyNode].MsgToBeVerified,EdDSA_INTERNAL[VerifyNode].MsgLastVerified,1) ,OTL(EdDSA_INTERNAL[VerifyNode].ProcessingRequired) ] ,OTU(EdDSA_INTERNAL[VerifyNode].VerificationInProgress) OTU(VerificationInProgress) ];
END_ROUTINE
